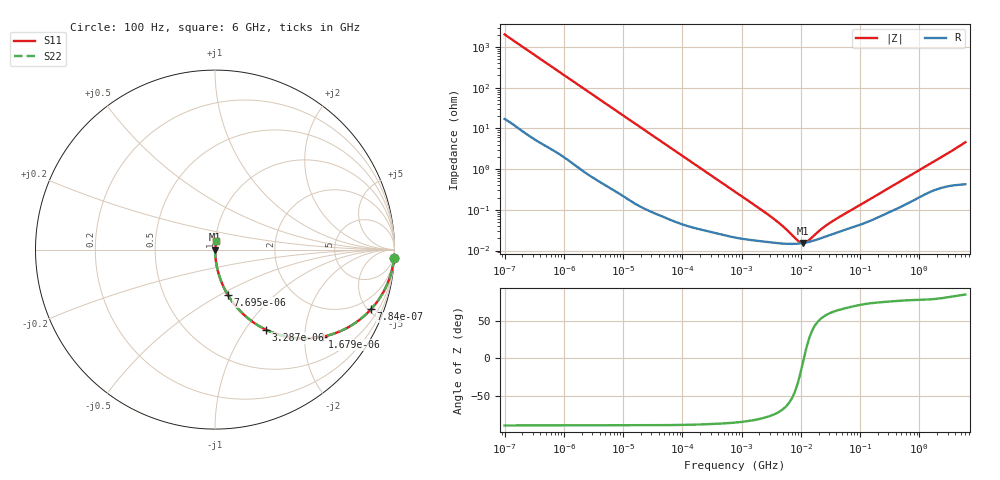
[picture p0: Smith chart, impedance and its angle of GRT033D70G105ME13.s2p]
!Murata Part Number: GRT033D70G105ME13
!These Parameters are Measured in Series Mode Connection
!Data Generated on Jun 19, 2026
!  o--ll--o
!Port1  Port2
!  o------o
!Operation Temp=25[degC], DC Bias Voltage=0[V]
!Freq. Start=100[Hz] Stop=6[GHz] 401[Steps]
# Hz S RI R 50
!Freq.(Hz) S11(Real) S11(Imag) S21(Real) S21(Imag) S12(Real) S12(Imag) S22(Real) S22(Imag)
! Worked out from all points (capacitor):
!   401 points, 100 Hz to 6 GHz, reference 50 ohm
!   read as one part in series: C = 784 nF near 109 Hz
!   lowest |Z| = 15.3 mohm at 10.87 MHz (marker M1)
!   series resonance near 11.27 MHz, so ESL is about 250 pH
!   S11 on the Smith chart (normalised r, x): 100 Hz: 1, -40; 784 Hz: 1.05, -5.22; 1.679 kHz: 1.02, -2.45; 3.287 kHz: 1.01, -1.26; 7.695 kHz: 1.01, -0.54; 6 GHz: 1.01, +0.09
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100  0.9972 -0.0492  0.00285 0.0492  0.00285 0.0492  0.9972 -0.0492
293  0.9786 -0.1405  0.0214 0.1405  0.0214 0.1405  0.9786 -0.1405
501  0.9414 -0.2305  0.0586 0.2305  0.0586 0.2305  0.9414 -0.2305
784  0.8698 -0.3318  0.1302 0.3318  0.1302 0.3318  0.8698 -0.3318
1174  0.7518 -0.4272  0.2482 0.4272  0.2482 0.4272  0.7518 -0.4272
1679  0.5996 -0.4854  0.4004 0.4854  0.4004 0.4854  0.5996 -0.4854
2008  0.5127 -0.4953  0.4873 0.4953  0.4873 0.4953  0.5127 -0.4953
3287  0.285 -0.4468  0.715 0.4468  0.715 0.4468  0.285 -0.4468
4918  0.153 -0.3551  0.847 0.3551  0.847 0.3551  0.153 -0.3551
7695  0.0701 -0.2502  0.9299 0.2502  0.9299 0.2502  0.0701 -0.2502
16473  0.0171 -0.1243  0.9829 0.1243  0.9829 0.1243  0.0171 -0.1243
40335  0.00343 -0.0517  0.9966 0.0517  0.9966 0.0517  0.00343 -0.0517
774597  0.000216 -0.00278  0.9998 0.00278  0.9998 0.00278  0.000216 -0.00278
3245845  0.000158 -0.000633  0.9998 0.000633  0.9998 0.000633  0.000158 -0.000633
5079039  0.000148 -0.000356  0.9999 0.000356  0.9999 0.000356  0.000148 -0.000356
8692127  0.000147 -0.000106  0.9999 0.000106  0.9999 0.000106  0.000147 -0.000106
1.087309e7  0.000153 -1.43e-05  0.9998 1.43e-05  0.9998 1.43e-05  0.000153 -1.43e-05
1.243624e7  0.000158 3.92e-05  0.9998 -3.92e-05  0.9998 -3.92e-05  0.000158 3.92e-05
1.555665e7  0.000171 0.000128  0.9998 -0.000128  0.9998 -0.000128  0.000171 0.000128
3.482834e7  0.000255 0.00047  0.9997 -0.00047  0.9997 -0.00047  0.000255 0.00047
3.124326e8  0.000886 0.00335  0.9991 -0.00335  0.9991 -0.00335  0.000886 0.00335
6e9  0.00628 0.0452  0.9937 -0.0452  0.9937 -0.0452  0.00628 0.0452
